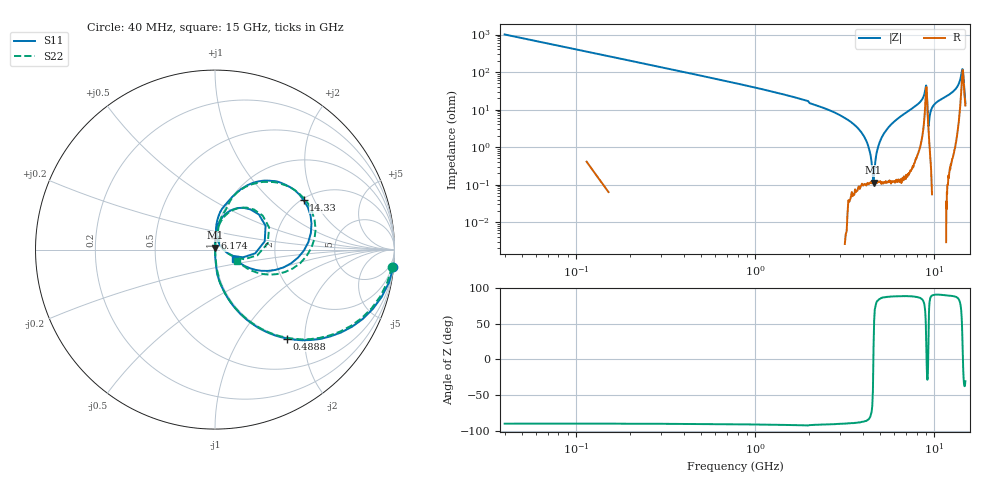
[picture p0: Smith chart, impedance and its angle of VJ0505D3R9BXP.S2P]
! VJ0505D3R9BXP
! MLCC placed on 25 mil thick microstrip substrate in series configuraton.
! DATE 06/29/2018  07:47
! CORRECTED  DATA
# GHz  S  MA  R  50.00
!  FREQ  S11M  S11A  S21M  S21A  S12M  S12A  S22M  S22A
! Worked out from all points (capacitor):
!   401 points, 40 MHz to 15 GHz, reference 50 ohm
!   read as one part in series: C = 3.94 pF near 114.8 MHz
!   lowest |Z| = 113 mohm at 4.603 GHz (marker M1)
!   series resonance near 4.594 GHz, so ESL is about 300 pH
!   S11 on the Smith chart (normalised r, x): 40 MHz: 0, -20; 488.8 MHz: 0.98, -1.64; 6.174 GHz: 0.99, +0.13; 14.33 GHz: 2.05, +1.66; 15 GHz: 1.24, -0.13
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0.04  0.9984 -5.7  0.09895 84.5  0.09854 84.7  0.9909 -5.6
0.227  0.8761 -29.4  0.491 60.9  0.4913 60.9  0.8686 -29.3
0.4888  0.6382 -50.9  0.7775 39.7  0.7782 39.7  0.6333 -50.8
1.1246  0.3227 -72.5  0.9544 19.1  0.9549 19.1  0.3212 -72.4
2.5458  0.09401 -86.1  0.9964 6.1  0.9969 6.1  0.09411 -84.9
3.8548  0.0189 -89.5  0.9982 2.1  0.9988 2.1  0.01884 -85.2
4.1166  0.008311 -89.5  0.9982 1.5  0.9988 1.5  0.008368 -79.5
4.3036  0.0008836 -110.5  0.9984 1.2  0.9987 1.1  0.001621 -19.7
4.3784  0.00191 94.4  0.9981 1.0  0.9986 1.0  0.002154 58.6
4.6028  0.01045 93.2  0.9983 0.5  0.9987 0.6  0.0104 80.4
5.0516  0.02654 91.1  0.9978 -0.3  0.9981 -0.3  0.02633 85.7
6.1736  0.06557 88.7  0.9957 -2.4  0.9966 -2.3  0.06545 84.9
7.52  0.1149 85.3  0.9897 -5.3  0.9904 -5.3  0.1175 82.2
9.016  0.3133 38.6  0.7643 -12.9  0.7647 -12.9  0.3264 35.6
9.3526  0.04282 61.2  0.9748 -0.9  0.9754 -0.9  0.04564 52.4
9.6144  0.1008 86.8  0.9912 -4.6  0.9915 -4.6  0.1032 80.7
10.0258  0.1426 86.7  0.9901 -7.0  0.9913 -7.0  0.146 80.9
12.5316  0.2681 75.7  0.9579 -14.9  0.9587 -14.9  0.2779 73.0
13.691  0.4032 63.1  0.8811 -23.3  0.8824 -23.3  0.4123 61.3
14.3268  0.5654 29.0  0.5535 -27.5  0.5538 -27.5  0.5799 25.4
14.6634  0.3936 -14.7  0.6261 10.8  0.6267 10.8  0.4096 -17.7
15  0.1216 -25.5  0.8843 4.0  0.885 4.0  0.1385 -26.1
